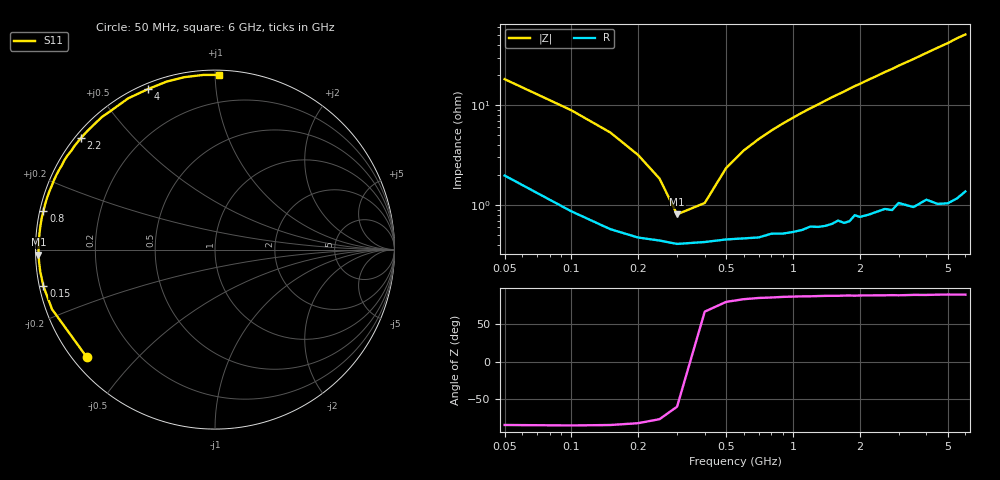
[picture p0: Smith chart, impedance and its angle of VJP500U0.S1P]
! Infineon Technologies  Discrete & RF Semiconductors
! BB 914
! Si Tuning Diode in SOT23
! VR = 0.5 V
! S-Parameters:  July  1999
# GHz  S  MA  R  50
!  f  S11
! GHz  MAG  ANG
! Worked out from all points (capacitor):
!   34 points, 50 MHz to 6 GHz, reference 50 ohm
!   read as one part to ground: C = 164 pF near 50 MHz
!   lowest |Z| = 809 mohm at 300 MHz (marker M1)
!   series resonance near 342.1 MHz, so ESL is about 1.3 nH
!   S11 on the Smith chart (normalised r, x): 50 MHz: 0.04, -0.36; 150 MHz: 0.01, -0.11; 800 MHz: 0.01, +0.11; 2.2 GHz: 0.02, +0.36; 4 GHz: 0.02, +0.67; 6 GHz: 0.03, +1.02
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0.05  0.9325 -140.1
0.1  0.9669 -159.9
0.15  0.9775 -167.9
0.2  0.9813 -172.8
0.25  0.9825 -175.9
0.3  0.9838 -178.4
0.4  0.9831 177.8
0.5  0.9821 174.7
0.6  0.9817 172.0
0.8  0.9798 167.3
1.1  0.9783 160.9
1.3  0.977 157.0
1.5  0.9757 153.0
1.6  0.974 151.2
1.8  0.9749 147.4
1.9  0.9715 145.5
2  0.9728 143.9
2.2  0.972 140.3
2.4  0.9706 137.0
2.6  0.9695 133.5
2.8  0.971 130.5
3  0.9669 127.1
3.5  0.9718 119.8
4  0.9691 112.6
4.5  0.9741 106.0
5  0.9758 100.1
5.5  0.9754 93.8
6  0.9735 88.8
